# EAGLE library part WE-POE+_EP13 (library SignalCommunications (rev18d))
Power over Ethernet Plus Transformer Characteristics Designed to meet 25 W PoE+ requirements of IEEE802.3at Frequency range: 250–400 kHz Input voltage range: 36–72 V 1.5 kV Hipot test between primary and secondary Operating temperature: –40 °C to +125 °C Applications PoE+ powered devices IP phones WLAN-Access points Security cameras Details see: http://katalog.we-online.de/en/pbs/WE-POE-PLUS?m Updated by Dan Xu 2014-07-08 2014 (C) Wurth Elektronik
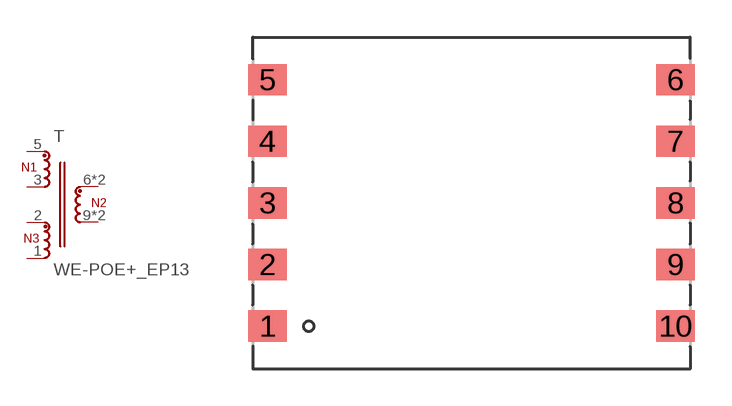
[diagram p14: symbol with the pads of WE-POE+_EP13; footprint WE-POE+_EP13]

Designator prefix T

## WE-POE+_EP13_750310743  [WE-POE+_EP13]
1  4  pas
2  5  pas
3  6  pas
5  1  pas
6  2  pas
7  2  pas
9  3  pas
10  3  pas

## WE-POE+_EP13_750310744  [WE-POE+_EP13]
Pads as for WE-POE+_EP13

## WE-POE+_EP13_750310742  [WE-POE+_EP13]
1  4  pas
2  5  pas
3  6  pas
5  1  pas
6  2  pas
10  3  pas

## Footprint WE-POE+_EP13 (pad centres in mm)
smd 1.55 x 1.27: 1 -8.275,-5; 2 -8.275,-2.5; 3 -8.275,0; 4 -8.275,2.5; 5 -8.275,5; 6 8.275,5; 7 8.275,2.5; 8 8.275,0; 9 8.275,-2.5; 10 8.275,-5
